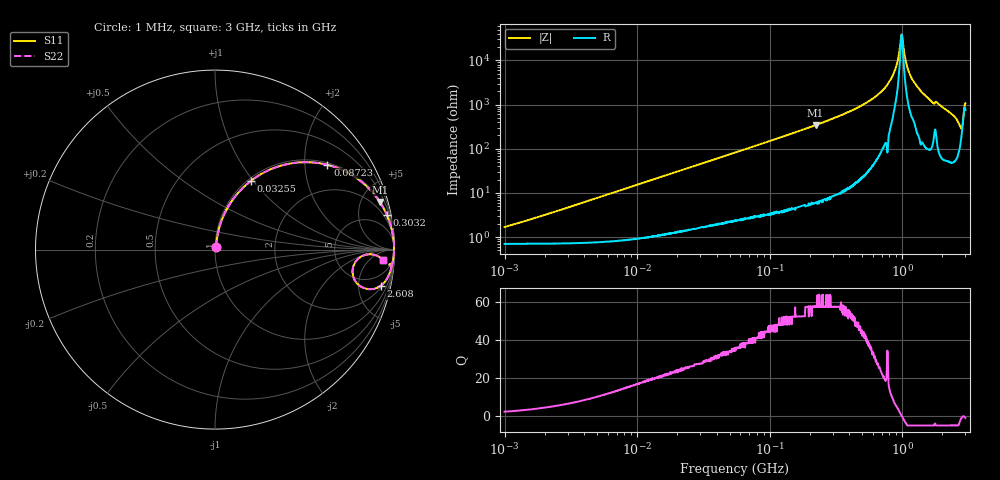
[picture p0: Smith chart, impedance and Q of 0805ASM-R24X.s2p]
!s-Parameter Generated by FASTRON Sdn. Bhd.
!FASTRON P/N : 0805ASM-R24X
!Keysight Technologies: E4991B_MY54100416_A.01.15
!Date: Fri Jun 19 14:51:17 2026
!Version  :Rev00  Fri Jun 19 14:51:17 2026
!Data & Calibration Information:
!Freq  S11  S21  S12  S22
!PortZ  Port1:50+j0  Port2:50+j0
!When reading reference impedance value at option line is always used.
! Remarks : This data is being provided solely for informational purposes.
# Hz S dB R 50
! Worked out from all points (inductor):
!   1601 points, 1 MHz to 3 GHz, reference 50 ohm
!   read as one part in series: L = 245 nH near 1.041 MHz
!   highest Q = 57.4 at 222.4 MHz (marker M1), where L = 246 nH
!   self-resonance near 987.8 MHz
!   S11 on the Smith chart (normalised r, x): 1 MHz: 1.01, +0.03; 32.55 MHz: 1.03, +0.98; 87.23 MHz: 1.06, +2.61; 303.2 MHz: 1.17, +9.79; 2.608 GHz: 2.28, -8.69; 3 GHz: 16, -15
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1000000  -35.50 64.7  -0.06 -0.9  -0.06 -0.9  -35.50 64.7
3804036  -24.70 79.5  -0.08 -3.3  -0.08 -3.3  -24.70 79.5
1.447069e7  -13.40 74.9  -0.29 -12.3  -0.29 -12.3  -13.40 74.9
3.254976e7  -7.25 62.3  -1.05 -25.7  -1.05 -25.7  -7.25 62.3
5.504702e7  -4.05 49.6  -2.37 -38.8  -2.37 -38.8  -4.05 49.6
8.723049e7  -2.11 37.0  -4.41 -51.6  -4.41 -51.6  -2.11 37.0
2.083556e8  -0.45 17.3  -10.60 -71.7  -10.60 -71.7  -0.45 17.3
2.223601e8  -0.39 16.1  -11.10 -72.9  -11.10 -72.9  -0.39 16.1
3.032461e8  -0.21 11.5  -14.00 -77.5  -14.00 -77.5  -0.21 11.5
5.668203e8  -0.05 4.7  -21.80 -83.8  -21.80 -83.8  -0.05 4.7
7.925923e8  -0.02 1.8  -30.20 -84.6  -30.20 -84.6  -0.02 1.8
8.892696e8  -0.02 0.9  -36.20 -79.5  -36.20 -79.5  -0.02 0.9
9.682285e8  -0.02 0.2  -47.30 -53.9  -47.30 -53.9  -0.02 0.2
9.977393e8  -0.02 -0.0  -51.50 16.6  -51.50 16.6  -0.02 -0.0
1.017911e9  -0.02 -0.2  -47.10 54.0  -47.10 54.0  -0.02 -0.2
1.113852e9  -0.03 -1.0  -35.50 79.3  -35.50 79.3  -0.03 -1.0
1.262285e9  -0.04 -2.0  -29.30 82.1  -29.30 82.1  -0.04 -2.0
1.67054e9  -0.10 -4.8  -21.50 80.0  -21.50 80.0  -0.10 -4.8
1.855641e9  -0.11 -5.2  -20.80 79.2  -20.80 79.2  -0.11 -5.2
2.607784e9  -0.49 -12.3  -13.30 69.3  -13.30 69.3  -0.49 -12.3
2.783064e9  -1.78 -13.5  -11.00 42.3  -11.00 42.3  -1.78 -13.5
3e9  -0.56 -3.6  -21.20 42.2  -21.20 42.2  -0.56 -3.6
